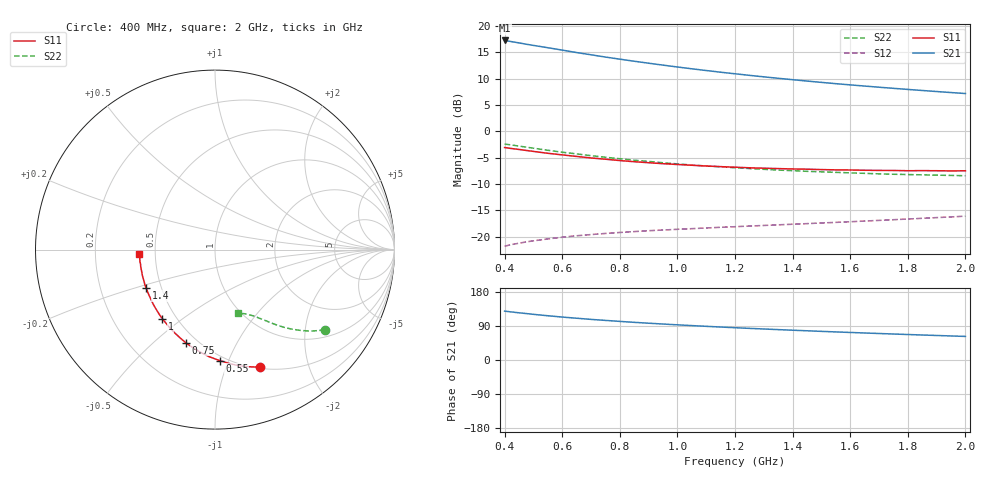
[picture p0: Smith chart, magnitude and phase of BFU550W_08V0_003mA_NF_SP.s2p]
! Filename:  P:\Prog\Test\Noise\ATS_data\Testdata_Net\06 Compressed Noise after Statistics\BFU550W_APM2013_11_D05_08p0V_003mA_NF_CM01_D.sf
! Date/Time: Tue 26/Mar/2013 16:25:23
! BFU550W_APM2013_11_D05_08p0V_1to35mA_NF_CM01_Bias3_R.sf
! Noise Parameter Data File
! BFU550W_APM2013_11_D05_08p0V_1to35mA_NF_CM01
! Date/time: Mon Mar 25 14:39:45 2013
! VAR V_out= 8.000000
! VAR I_out= 3.000000
! VAR V_in= 0.796400
! VAR I_in= 0.029610
! Device data file deembeded for feedlines and parallel
! Original file: \06 Compressed Noise after Statistics\BFU550W_APM2013_11_D05_08p0V_003mA_NF_CM01_R.sf
! Feed-files: PR019V01_070313_Feed1.s2p, PR019V01_070313_Feed2.s2p
! Parallel-file: PR019V01_070313_Par.s2p
# MHz S MA R 50
!  Freq-MHz  S11-mag  S11-arg  S21-mag  S21-arg  S12-mag  S12-arg  S22-mag  S22-arg
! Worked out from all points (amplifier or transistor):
!   37 points, 400 MHz to 2 GHz, reference 50 ohm
!   highest |S21| = 17.2 dB at 400 MHz (marker M1)
!   |S21| within 3 dB of that: start of sweep to 733 MHz
!   unconditionally stable (mu >= 1): 1.961 GHz to end of sweep
!   at 500 MHz: K = 0.37, MSG = 18.5 dB, |S12| = -20.8 dB
!   at 1.1 GHz: K = 0.72, MSG = 14.9 dB, |S12| = -18.3 dB
!   at 2 GHz: K = 1.00, MAG = 11.2 dB, |S12| = -16.1 dB
!   lowest NFmin = 0.47 dB at 420 MHz
!   S11 on the Smith chart (normalised r, x): 400 MHz: 0.51, -1.32; 550 MHz: 0.46, -0.93; 750 MHz: 0.43, -0.64; 1 GHz: 0.42, -0.42; 1.4 GHz: 0.41, -0.22; 2 GHz: 0.41, -0.02
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400  0.7008 -69.0  7.265 128.9  0.08136 55.5  0.7572 -36.0
420  0.6885 -71.8  7.114 127.1  0.0837 54.5  0.7437 -37.1
440  0.6775 -74.4  6.963 125.4  0.08585 53.6  0.7304 -38.1
480  0.6554 -79.3  6.656 122.2  0.08969 51.9  0.7039 -40.1
500  0.6441 -81.9  6.523 120.5  0.09144 51.1  0.6913 -41.0
550  0.6186 -87.7  6.199 116.8  0.09529 49.5  0.6605 -43.1
600  0.5972 -93.2  5.886 113.3  0.09888 48.1  0.6331 -44.8
650  0.5772 -98.1  5.578 110.2  0.1021 47.0  0.6102 -46.4
700  0.5584 -103.2  5.315 107.2  0.1048 46.0  0.587 -47.9
750  0.5434 -107.6  5.057 104.5  0.1074 45.3  0.5671 -49.1
800  0.5275 -112.0  4.829 101.9  0.1097 44.7  0.5488 -50.4
850  0.5146 -116.2  4.616 99.4  0.1119 44.2  0.5318 -51.4
950  0.4927 -123.7  4.239 94.9  0.1158 43.7  0.5028 -53.4
1000  0.4842 -127.3  4.07 92.8  0.1176 43.6  0.4905 -54.2
1100  0.4686 -133.8  3.768 88.9  0.1211 43.6  0.4684 -55.9
1200  0.4564 -139.9  3.509 85.2  0.1245 43.8  0.4509 -57.6
1300  0.4465 -145.7  3.282 81.8  0.1279 44.2  0.4357 -59.0
1400  0.4391 -150.9  3.084 78.6  0.1313 44.9  0.4231 -60.4
1500  0.4333 -155.9  2.909 75.6  0.135 45.5  0.4125 -62.0
1600  0.4294 -160.5  2.755 72.7  0.1387 46.4  0.4031 -63.5
1750  0.4249 -166.8  2.555 68.6  0.145 47.7  0.3913 -65.7
2000  0.422 -176.6  2.28 62.2  0.1567 49.8  0.3789 -69.8
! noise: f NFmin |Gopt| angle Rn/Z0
400  0.5358  0.3584  34.57  0.1268
460  0.5308  0.3567  39.04  0.1321
600  0.5934  0.3468  49.23  0.1326
800  0.6215  0.3463  65.75  0.1188
1000  0.6972  0.3526  78.64  0.1144
1200  0.7152  0.3598  93.69  0.1063
1400  0.763  0.3676  110.5  0.0925
1600  0.7437  0.3971  122.6  0.0776
1800  0.8895  0.4031  138.2  0.0651
2000  0.9037  0.4193  150.6  0.059
